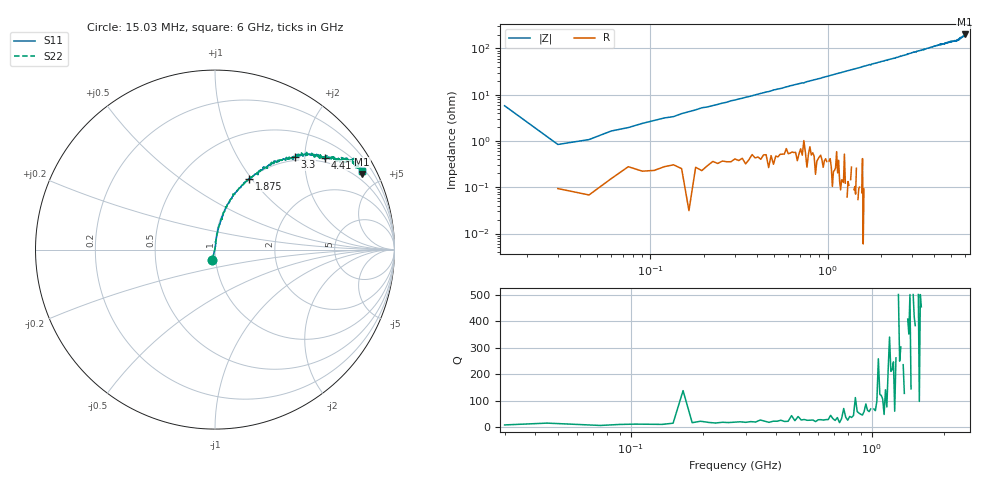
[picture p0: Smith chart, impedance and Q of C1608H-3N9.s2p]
!	Network	Analyzer	HP8753E.07.74:	Oct	30	2002	Serial	No.	JP38451487
!	Hewlett-Packard
!	7	Sep	2009	10:12:05
!	Frequency	S11	S21	S12	S22
#	HZ	S	RI	R	50
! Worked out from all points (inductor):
!   400 points, 15.03 MHz to 6 GHz, reference 50 ohm
!   read as one part in series: L = 4.1 nH near 45.03 MHz
!   highest |Z| = 201 ohm at 5.955 GHz (marker M1)
!   S11 on the Smith chart (normalised r, x): 15.03 MHz: 0.96, -0.11; 1.875 GHz: 0.99, +0.97; 3.3 GHz: 0.93, +1.79; 4.41 GHz: 0.88, +2.48; 6 GHz: 0.61, +3.91
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1.502992e7  -0.0151 -0.0562  1.02 0.0562  1.02 0.0562  -0.0151 -0.0562
3.002985e7  0.00101 0.00835  0.999 -0.00835  0.999 -0.00835  0.00101 0.00835
4.502978e7  0.000591 0.0107  0.999 -0.0107  0.999 -0.0107  0.000591 0.0107
6.00297e7  0.00159 0.0163  0.998 -0.0163  0.998 -0.0163  0.00159 0.0163
1.050295e8  0.00313 0.0275  0.997 -0.0275  0.997 -0.0275  0.00313 0.0275
1.95029e8  0.00496 0.0518  0.995 -0.0518  0.995 -0.0518  0.00496 0.0518
2.850286e8  0.00889 0.0731  0.991 -0.0731  0.991 -0.0731  0.00889 0.0731
6.150269e8  0.0288 0.151  0.971 -0.151  0.971 -0.151  0.0288 0.151
1.020025e9  0.0644 0.238  0.936 -0.238  0.936 -0.238  0.0644 0.238
1.875021e9  0.189 0.396  0.811 -0.396  0.811 -0.396  0.189 0.396
2.01002e9  0.213 0.411  0.787 -0.411  0.787 -0.411  0.213 0.411
3.015015e9  0.398 0.513  0.602 -0.513  0.602 -0.513  0.398 0.513
3.300014e9  0.443 0.517  0.557 -0.517  0.557 -0.517  0.443 0.517
4.00501e9  0.567 0.531  0.433 -0.531  0.433 -0.531  0.567 0.531
4.410008e9  0.611 0.513  0.389 -0.513  0.389 -0.513  0.611 0.513
5.010005e9  0.675 0.501  0.325 -0.501  0.325 -0.501  0.675 0.501
5.535002e9  0.719 0.485  0.281 -0.485  0.281 -0.485  0.719 0.485
5.565002e9  0.776 0.508  0.224 -0.508  0.224 -0.508  0.776 0.508
5.595002e9  0.744 0.494  0.256 -0.494  0.256 -0.494  0.744 0.494
5.625002e9  0.785 0.486  0.215 -0.486  0.215 -0.486  0.785 0.486
5.955e9  0.82 0.422  0.18 -0.422  0.18 -0.422  0.82 0.422
6e9  0.82 0.438  0.18 -0.438  0.18 -0.438  0.82 0.438
